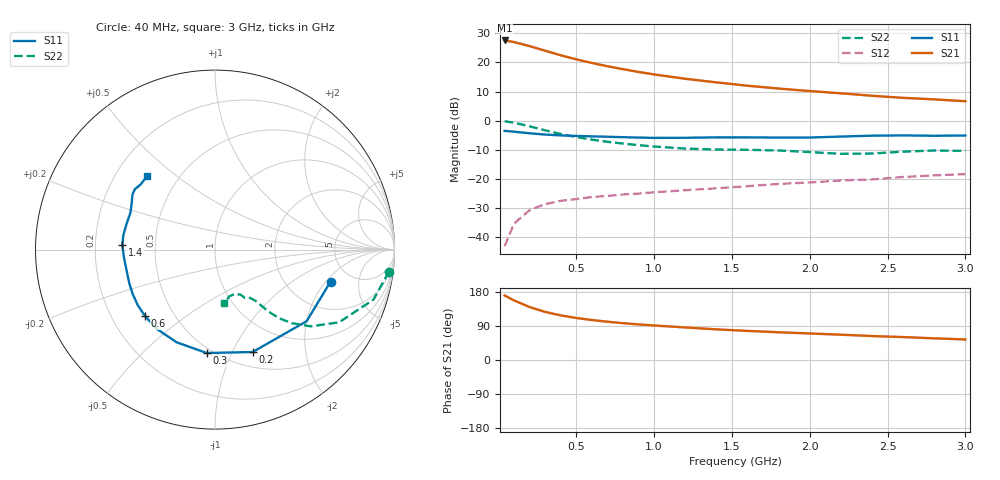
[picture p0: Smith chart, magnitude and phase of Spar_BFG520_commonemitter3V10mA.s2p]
! Filename:  BFG520C.S2P  Version:  2.1
! NXP part #: BFG520  Date: Feb 1992
! Bias condition: Vce=3V, Ic=10mA
! IN LINE PINNING: same data as with cross emitter pinning.
#  MHz  S  MA  R  50
! Freq  S11  S21  S12  S22  !GUM [dB]
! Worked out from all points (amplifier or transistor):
!   21 points, 40 MHz to 3 GHz, reference 50 ohm
!   highest |S21| = 27.6 dB at 40 MHz (marker M1)
!   |S21| within 3 dB of that: start of sweep to 267.5 MHz
!   unconditionally stable (mu >= 1): 1.261 GHz to end of sweep
!   at 300 MHz: K = 0.32, MSG = 26.3 dB, |S12| = -28.6 dB
!   at 1 GHz: K = 0.88, MSG = 20.2 dB, |S12| = -24.6 dB
!   at 3 GHz: K = 1.26, MAG = 9.5 dB, |S12| = -18.3 dB
!   lowest NFmin = 1.10 dB at 500 MHz
!   S11 on the Smith chart (normalised r, x): 40 MHz: 3.49, -2.25; 200 MHz: 0.66, -1.20; 300 MHz: 0.47, -0.81; 600 MHz: 0.34, -0.36; 1.4 GHz: 0.32, +0.02; 3 GHz: 0.33, +0.40
40  0.668 -15.5  23.88 170.3  0.007 81.8  0.977 -7.2
100  0.648 -38.0  22.43 157.3  0.017 73.4  0.926 -17.5
200  0.608 -69.8  19.09 139.8  0.029 61.1  0.801 -30.4
300  0.578 -94.6  15.94 126.9  0.037 53.9  0.684 -38.7
400  0.559 -112.5  13.29 117.8  0.042 50.3  0.592 -43.8
500  0.548 -126.0  11.32 110.9  0.045 47.5  0.524 -46.9
600  0.538 -136.3  9.809 105.5  0.049 46.9  0.473 -48.6
700  0.53 -144.3  8.626 101.0  0.051 47.1  0.434 -49.7
800  0.521 -151.7  7.669 97.2  0.054 47.8  0.405 -50.4
900  0.513 -158.5  6.874 93.9  0.056 49.0  0.38 -51.1
1000  0.507 -164.4  6.235 91.1  0.059 50.2  0.36 -51.9
1200  0.509 -174.9  5.249 85.9  0.064 51.5  0.332 -54.1
1400  0.517 177.1  4.552 80.9  0.069 53.0  0.32 -56.9
1600  0.517 170.7  3.987 76.8  0.075 56.2  0.316 -58.3
1800  0.513 163.7  3.566 73.2  0.082 57.1  0.308 -58.9
2000  0.514 156.4  3.228 70.0  0.087 59.0  0.289 -60.4
2200  0.534 150.2  2.952 66.8  0.094 59.6  0.27 -65.9
2400  0.553 146.2  2.68 63.2  0.098 61.3  0.273 -73.3
2600  0.559 143.0  2.469 60.5  0.108 61.9  0.294 -78.0
2800  0.551 138.8  2.324 57.2  0.115 61.5  0.308 -79.1
3000  0.557 132.8  2.162 54.2  0.121 62.8  0.302 -80.1
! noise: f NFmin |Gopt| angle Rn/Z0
500  1.1  0.26  27  0.22
900  1.25  0.231  54  0.22
1000  1.3  0.24  58  0.24
2000  1.9  0.245  148  0.14
